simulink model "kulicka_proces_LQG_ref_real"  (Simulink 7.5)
libraries: mathlib x38, execlib x4, reglib x4, inoutlib x2, anallib x1, arclib x1

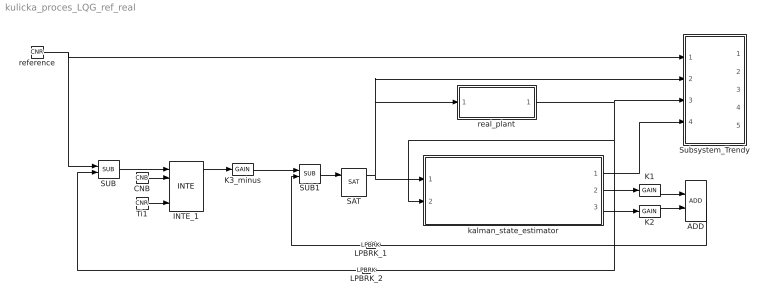
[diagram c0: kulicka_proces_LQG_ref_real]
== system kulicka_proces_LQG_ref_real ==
  ADD : mathlib/ADD  SystemSampleTime=-1
  CNB : mathlib/CNB  SystemSampleTime=-1  YCN=on
  INTE_1 : anallib/INTE  ymin=-1  ymax=1
  K1 : mathlib/GAIN  SystemSampleTime=-1  k=1.491313
  K2 : mathlib/GAIN  SystemSampleTime=-1  k=1.11034
  K3_minus : mathlib/GAIN  SystemSampleTime=-1  k=0.057735
  LPBRK_1 : execlib/LPBRK  Orientation=left
  LPBRK_2 : execlib/LPBRK  Orientation=left
  SAT : reglib/SAT  SystemSampleTime=-1  tp=1  tn=1  hilim0=0.01  lolim0=-0.01  HLD=on
  SUB : mathlib/SUB  SystemSampleTime=-1
  SUB1 : mathlib/SUB  SystemSampleTime=-1
  Subsystem_Trendy : Subsystem
  Ti1 : mathlib/CNR  SystemSampleTime=-1  ycn=1
  kalman_state_estimator : Subsystem
  real_plant : Subsystem
  reference : mathlib/CNR  SystemSampleTime=-1  ycn=0.5
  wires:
  ADD/1 -> LPBRK_1/1
  CNB/1 -> INTE_1/2
  INTE_1/1 -> K3_minus/1
  K1/1 -> ADD/1
  K2/1 -> ADD/2
  K3_minus/1 -> SUB1/1
  LPBRK_1/1 -> SUB1/2
  LPBRK_2/1 -> SUB/2
  SAT/1 -> kalman_state_estimator/1(u), Subsystem_Trendy/2(u_out), real_plant/1(u)
  SUB/1 -> INTE_1/1
  SUB1/1 -> SAT/1
  Ti1/1 -> INTE_1/5
  kalman_state_estimator/1(y_kalman) -> Subsystem_Trendy/4(y_est)
  kalman_state_estimator/2(x1_kalman) -> K1/1
  kalman_state_estimator/3(x2_kalman) -> K2/1
  real_plant/1(y) -> Subsystem_Trendy/3(y_out), LPBRK_2/1, kalman_state_estimator/2(y)
  reference/1 -> SUB/1, Subsystem_Trendy/1(w_in)

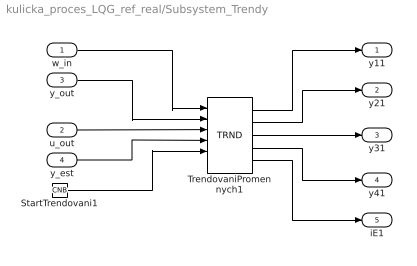
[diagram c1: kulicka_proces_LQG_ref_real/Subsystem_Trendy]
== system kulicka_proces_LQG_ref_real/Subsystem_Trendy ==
  w_in : Inport  Port=1
  u_out : Inport  Port=2
  y_out : Inport  Port=3
  y_est : Inport  Port=4
  StartTrendovani1 : mathlib/CNB  SystemSampleTime=-1  YCN=on
  TrendovaniPromennych1 : arclib/TRND  SystemSampleTime=-1  n=4  l=1000  btype=8: Double  ptype1=1: Store  ptype2=1: Store  ptype3=1: Store  ptype4=1: Store  pfac=1  afac=0  arc=2  id=1  Title=Trend Title
  y11 : Outport  Port=1
  y21 : Outport  Port=2
  y31 : Outport  Port=3
  y41 : Outport  Port=4
  iE1 : Outport  Port=5
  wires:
  StartTrendovani1/1 -> TrendovaniPromennych1/5
  TrendovaniPromennych1/1 -> y11/1
  TrendovaniPromennych1/2 -> y21/1
  TrendovaniPromennych1/3 -> y31/1
  TrendovaniPromennych1/4 -> y41/1
  TrendovaniPromennych1/5 -> iE1/1
  u_out/1 -> TrendovaniPromennych1/3
  w_in/1 -> TrendovaniPromennych1/1
  y_est/1 -> TrendovaniPromennych1/4
  y_out/1 -> TrendovaniPromennych1/2

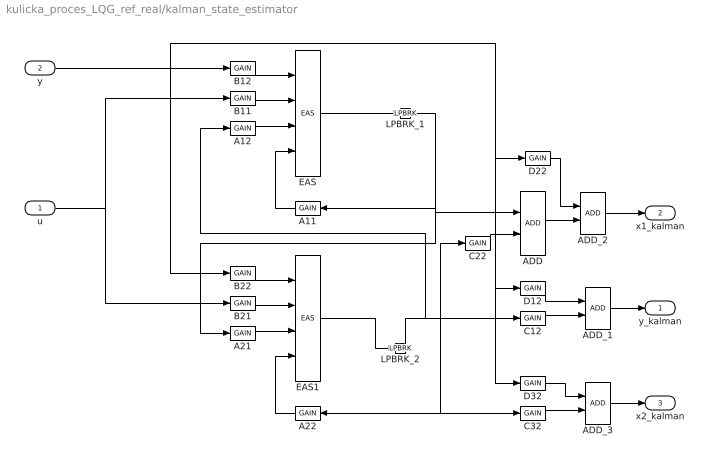
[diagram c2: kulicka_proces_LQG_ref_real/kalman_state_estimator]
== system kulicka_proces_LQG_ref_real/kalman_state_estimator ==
  u : Inport  Port=1
  y : Inport  Port=2
  A11 : mathlib/GAIN  Orientation=left  SystemSampleTime=-1  k=1
  A12 : mathlib/GAIN  SystemSampleTime=-1  k=-0.137504
  A21 : mathlib/GAIN  SystemSampleTime=-1  k=0.02
  A22 : mathlib/GAIN  Orientation=left  SystemSampleTime=-1  k=0.924458
  ADD : mathlib/ADD  SystemSampleTime=-1
  ADD_1 : mathlib/ADD  SystemSampleTime=-1
  ADD_2 : mathlib/ADD  SystemSampleTime=-1
  ADD_3 : mathlib/ADD  SystemSampleTime=-1
  B11 : mathlib/GAIN  SystemSampleTime=-1  k=0.02
  B12 : mathlib/GAIN  SystemSampleTime=-1  k=0.019258
  B21 : mathlib/GAIN  SystemSampleTime=-1  k=0.0002
  B22 : mathlib/GAIN  SystemSampleTime=-1  k=0.01058
  C12 : mathlib/GAIN  SystemSampleTime=-1  k=6.620262
  C22 : mathlib/GAIN  SystemSampleTime=-1  k=-0.137504
  C32 : mathlib/GAIN  SystemSampleTime=-1  k=0.927208
  D12 : mathlib/GAIN  SystemSampleTime=-1  k=0.072792
  D22 : mathlib/GAIN  SystemSampleTime=-1  k=0.019258
  D32 : mathlib/GAIN  SystemSampleTime=-1  k=0.010195
  EAS : mathlib/EAS  SystemSampleTime=-1  a=1  b=1  c=1  d=1  y0=0
  EAS1 : mathlib/EAS  SystemSampleTime=-1  a=1  b=1  c=1  d=1  y0=0
  LPBRK_1 : execlib/LPBRK
  LPBRK_2 : execlib/LPBRK
  y_kalman : Outport  Port=1
  x1_kalman : Outport  Port=2
  x2_kalman : Outport  Port=3
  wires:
  A11/1 -> EAS/4
  A12/1 -> EAS/3
  A21/1 -> EAS1/3
  A22/1 -> EAS1/4
  ADD/1 -> ADD_2/2
  ADD_1/1 -> y_kalman/1
  ADD_2/1 -> x1_kalman/1
  ADD_3/1 -> x2_kalman/1
  B11/1 -> EAS/2
  B12/1 -> EAS/1
  B21/1 -> EAS1/2
  B22/1 -> EAS1/1
  C12/1 -> ADD_1/2
  C22/1 -> ADD/2
  C32/1 -> ADD_3/2
  D12/1 -> ADD_1/1
  D22/1 -> ADD_2/1
  D32/1 -> ADD_3/1
  EAS/1 -> LPBRK_1/1
  EAS1/1 -> LPBRK_2/1
  LPBRK_1/1 -> A11/1, A21/1, ADD/1
  LPBRK_2/1 -> A12/1, C12/1, C22/1, A22/1, C32/1
  u/1 -> B11/1, B21/1
  y/1 -> B12/1, B22/1, D22/1, D12/1, D32/1

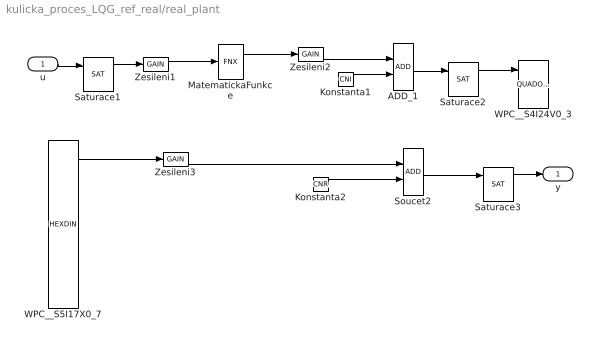
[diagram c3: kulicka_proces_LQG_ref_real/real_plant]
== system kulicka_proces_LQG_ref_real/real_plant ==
  u : Inport  Port=1
  ADD_1 : mathlib/ADD  SystemSampleTime=-1
  Konstanta1 : mathlib/CNI  SystemSampleTime=-1  ycn=5
  Konstanta2 : mathlib/CNR  SystemSampleTime=-1  ycn=0.96
  MatematickaFunkce : mathlib/FNX  SystemSampleTime=-1  ifn=2: asin  yerr=0
  Saturace1 : reglib/SAT  SystemSampleTime=-1  tp=1  tn=1  hilim0=0.01  lolim0=-0.01  HLD=on
  Saturace2 : reglib/SAT  SystemSampleTime=-1  tp=1  tn=1  hilim0=10  lolim0=0  HLD=on
  Saturace3 : reglib/SAT  SystemSampleTime=-1  tp=1  tn=1  hilim0=0.95  lolim0=0  HLD=on
  Soucet2 : mathlib/ADD  SystemSampleTime=-1
  WPC__S4I24V0_3 : inoutlib/QUADOUT  SystemSampleTime=-1
  WPC__S5I17X0_7 : inoutlib/HEXDIN  SystemSampleTime=-1
  Zesileni1 : mathlib/GAIN  SystemSampleTime=-1  k=50
  Zesileni2 : mathlib/GAIN  SystemSampleTime=-1  k=9.5493
  Zesileni3 : mathlib/GAIN  SystemSampleTime=-1  k=-0.1
  y : Outport  Port=1
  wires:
  ADD_1/1 -> Saturace2/1
  Konstanta1/1 -> ADD_1/2
  Konstanta2/1 -> Soucet2/2
  MatematickaFunkce/1 -> Zesileni2/1
  Saturace1/1 -> Zesileni1/1
  Saturace2/1 -> WPC__S4I24V0_3/1
  Saturace3/1 -> y/1
  Soucet2/1 -> Saturace3/1
  WPC__S5I17X0_7/2 -> Zesileni3/1
  Zesileni1/1 -> MatematickaFunkce/1
  Zesileni2/1 -> ADD_1/1
  Zesileni3/1 -> Soucet2/1
  u/1 -> Saturace1/1
